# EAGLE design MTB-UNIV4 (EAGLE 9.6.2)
Assembly variants: PFH, SVORK
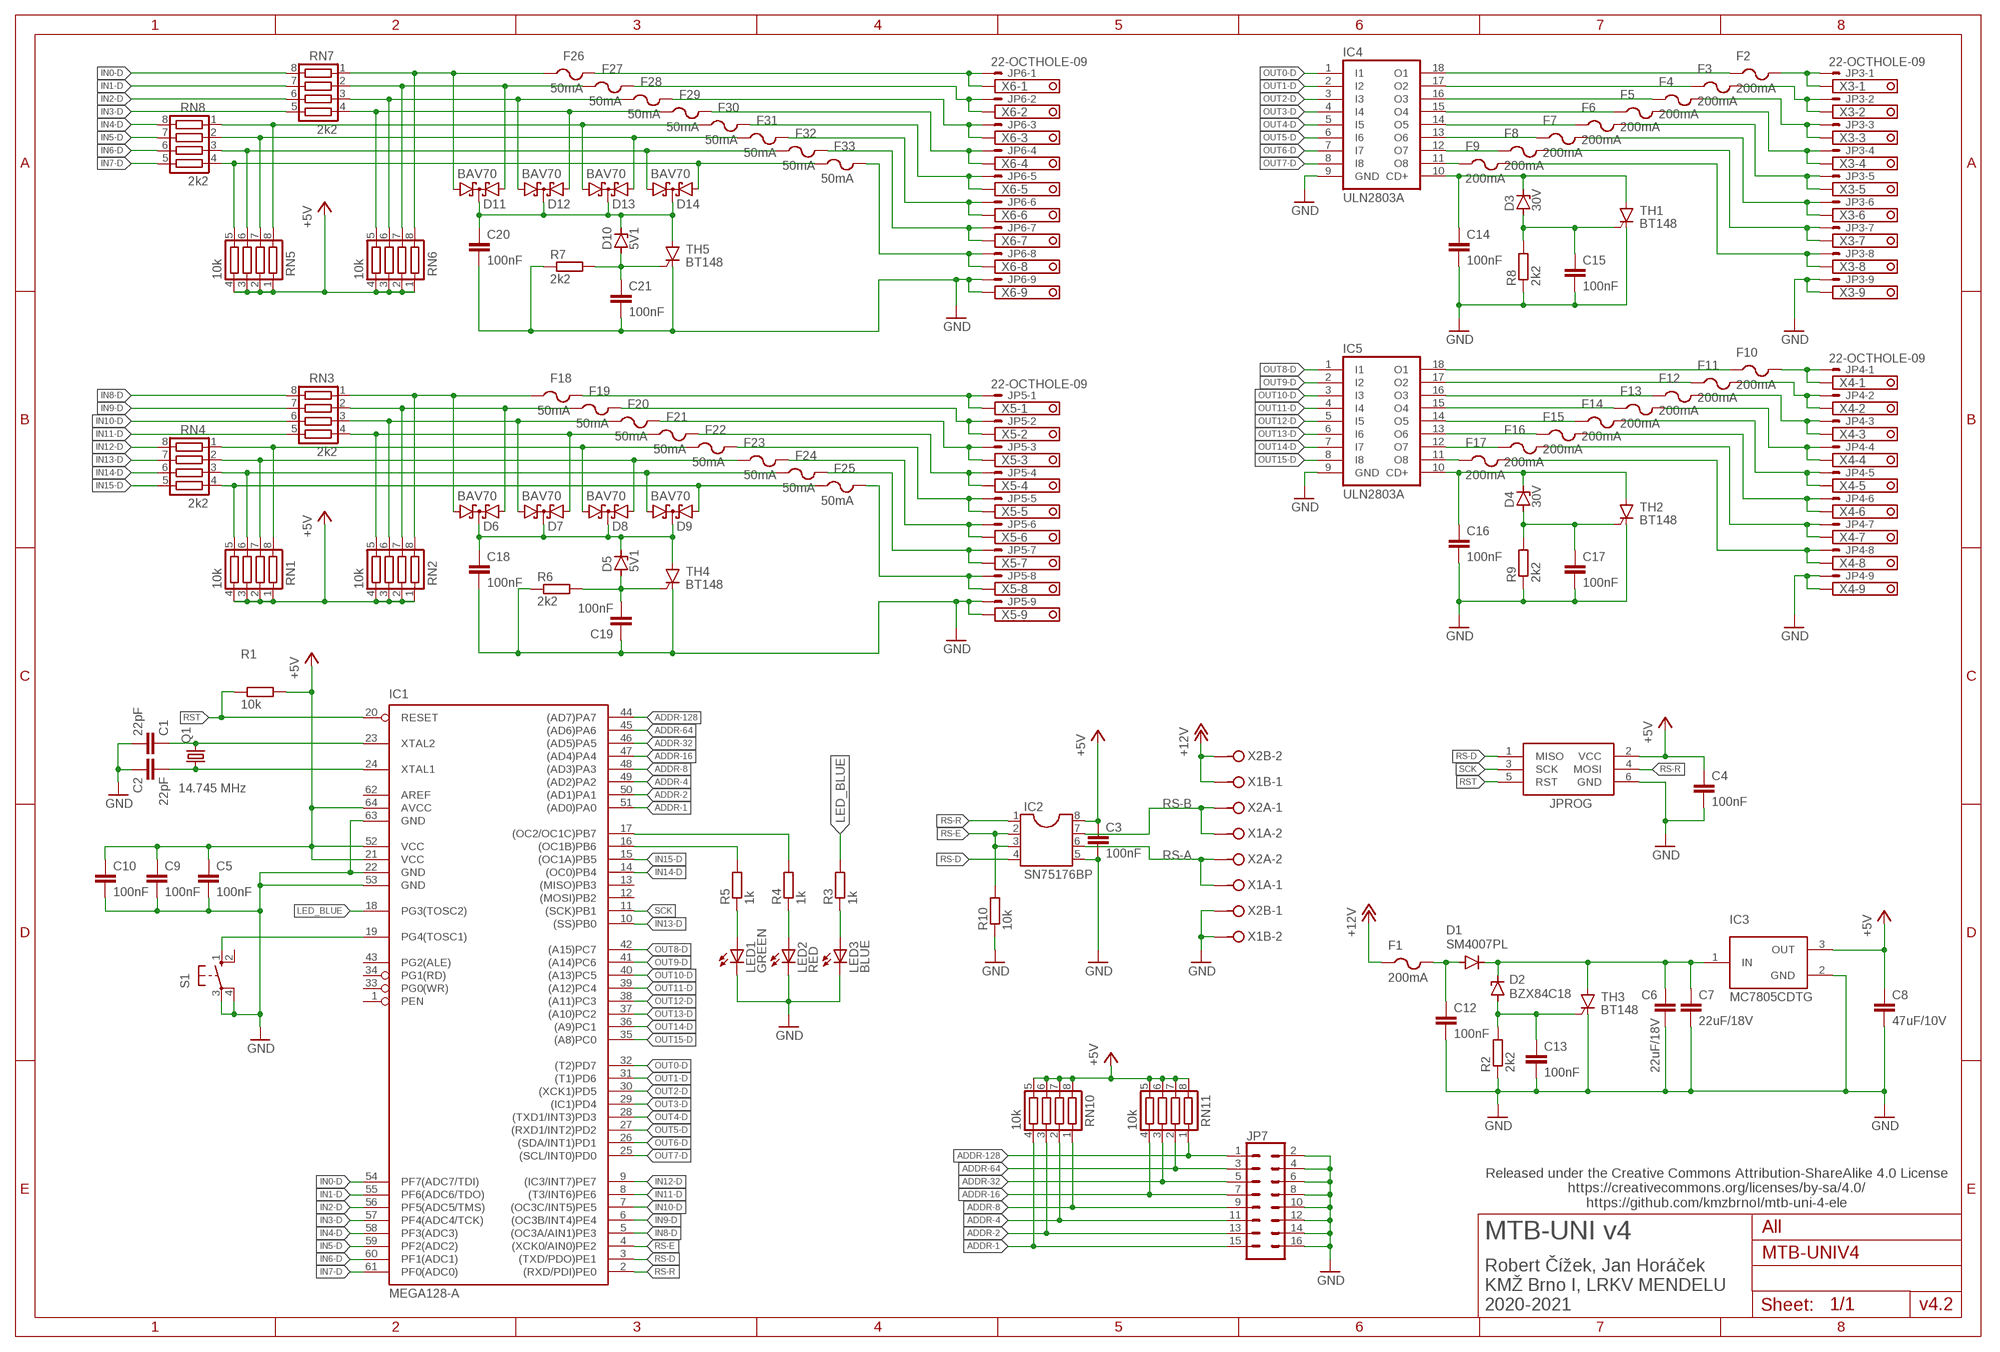
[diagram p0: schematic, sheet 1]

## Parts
C1  22pF  C-EUC0805  [C0805]
C2  22pF  C-EUC0805  [C0805]
C3  100nF  C-EUC0805  [C0805]
C4  100nF  C-EUC0805  [C0805]
C5  100nF  C-EUC0805  [C0805]
C6  22uF/18V  C-EUC0805  [C0805]
C7  22uF/18V  C-EUC1206  [C1206]
C8  47uF/10V  C-EUC1206  [C1206]
C9  100nF  C-EUC0805  [C0805]
C10  100nF  C-EUC0805  [C0805]
C12  100nF  C-EUC0805  [C0805]
C13  100nF  C-EUC0805  [C0805]
C14  100nF  C-EUC0805  [C0805]
C15  100nF  C-EUC0805  [C0805]
C16  100nF  C-EUC0805  [C0805]
C17  100nF  C-EUC0805  [C0805]
C18  100nF  C-EUC0805  [C0805]
C19  100nF  C-EUC0805  [C0805]
C20  100nF  C-EUC0805  [C0805]
C21  100nF  C-EUC0805  [C0805]
D1  SM4007PL  CGRM4007-G  [SOD-123_MINI-SMA]
D2  BZX84C18  ZENER-DIODESOT23  [SOT23]
D3  30V  ZENER-DIODESOT23  [SOT23]
D4  30V  ZENER-DIODESOT23  [SOT23]
D5  5V1  ZENER-DIODESOT23  [SOT23]
D6  BAV70  BAT54C  [SOT23]
D7  BAV70  BAT54C  [SOT23]
D8  BAV70  BAT54C  [SOT23]
D9  BAV70  BAT54C  [SOT23]
D10  5V1  ZENER-DIODESOT23  [SOT23]
D11  BAV70  BAT54C  [SOT23]
D12  BAV70  BAT54C  [SOT23]
D13  BAV70  BAT54C  [SOT23]
D14  BAV70  BAT54C  [SOT23]
F1  200mA  PTCFUSE-1206  [R1206]
F2  200mA  PTCFUSE-1206S  [R1206S]
F3  200mA  PTCFUSE-1206S  [R1206S]
F4  200mA  PTCFUSE-1206S  [R1206S]
F5  200mA  PTCFUSE-1206S  [R1206S]
F6  200mA  PTCFUSE-1206S  [R1206S]
F7  200mA  PTCFUSE-1206S  [R1206S]
F8  200mA  PTCFUSE-1206S  [R1206S]
F9  200mA  PTCFUSE-1206S  [R1206S]
F10  200mA  PTCFUSE-1206S  [R1206S]
F11  200mA  PTCFUSE-1206S  [R1206S]
F12  200mA  PTCFUSE-1206S  [R1206S]
F13  200mA  PTCFUSE-1206S  [R1206S]
F14  200mA  PTCFUSE-1206S  [R1206S]
F15  200mA  PTCFUSE-1206S  [R1206S]
F16  200mA  PTCFUSE-1206S  [R1206S]
F17  200mA  PTCFUSE-1206S  [R1206S]
F18  50mA  PTCFUSE-1206S  [R1206S]
F19  50mA  PTCFUSE-1206S  [R1206S]
F20  50mA  PTCFUSE-1206S  [R1206S]
F21  50mA  PTCFUSE-1206S  [R1206S]
F22  50mA  PTCFUSE-1206S  [R1206S]
F23  50mA  PTCFUSE-1206S  [R1206S]
F24  50mA  PTCFUSE-1206S  [R1206S]
F25  50mA  PTCFUSE-1206S  [R1206S]
F26  50mA  PTCFUSE-1206S  [R1206S]
F27  50mA  PTCFUSE-1206S  [R1206S]
F28  50mA  PTCFUSE-1206S  [R1206S]
F29  50mA  PTCFUSE-1206S  [R1206S]
F30  50mA  PTCFUSE-1206S  [R1206S]
F31  50mA  PTCFUSE-1206S  [R1206S]
F32  50mA  PTCFUSE-1206S  [R1206S]
F33  50mA  PTCFUSE-1206S  [R1206S]
IC1  MEGA128-A  [TQFP64]
IC2  SN75176BP  DIL8  [DIL08]
IC3  MC7805CDTG  MC78M05BDTRKG  [MC78M05BDTRKG]
IC4  ULN2803A  [DIL18]
IC5  ULN2803A  [DIL18]
JP3  22-OCTHOLE-09  [7395-09-OCTHOLE]  (not fitted in variant SVORK)
JP4  22-OCTHOLE-09  [7395-09-OCTHOLE]  (not fitted in variant SVORK)
JP5  22-OCTHOLE-09  [7395-09-OCTHOLE]  (not fitted in variant SVORK)
JP6  22-OCTHOLE-09  [7395-09-OCTHOLE]  (not fitted in variant SVORK)
JP7  CONN_08X2  [2X8]
JPROG  AVRISP-6  [AVRISP]
LED1  GREEN  LEDCHIPLED_0805  [CHIPLED_0805]
LED2  RED  LEDCHIPLED_0805  [CHIPLED_0805]
LED3  BLUE  LEDCHIPLED_0805  [CHIPLED_0805]
Q1  14.745 MHz  CRYSTALHC49UP  [HC49UP]
R1  10k  R-EU_R0805  [R0805]
R2  2k2  R-EU_R0805  [R0805]
R3  1k  R-EU_R0805  [R0805]
R4  1k  R-EU_R0805  [R0805]
R5  1k  R-EU_R0805  [R0805]
R6  2k2  R-EU_R0805  [R0805]
R7  2k2  R-EU_R0805  [R0805]
R8  2k2  R-EU_R0805  [R0805]
R9  2k2  R-EU_R0805  [R0805]
R10  10k  R-EU_R0805  [R0805]
RN1  10k  CTS742C083  [CTS742C083]
RN2  10k  CTS742C083  [CTS742C083]
RN3  2k2  CTS742C083  [CTS742C083]
RN4  2k2  CTS742C083  [CTS742C083]
RN5  10k  CTS742C083  [CTS742C083]
RN6  10k  CTS742C083  [CTS742C083]
RN7  2k2  CTS742C083  [CTS742C083]
RN8  2k2  CTS742C083  [CTS742C083]
RN10  10k  CTS742C083  [CTS742C083]
RN11  10k  CTS742C083  [CTS742C083]
S1  10-XX  [B3F-10XX]
TH1  BT148  [SOT223]
TH2  BT148  [SOT223]
TH3  BT148  [SOT223]
TH4  BT148  [SOT223]
TH5  BT148  [SOT223]
X1A  MVE252-5-V  [MVE252-5-V]
X1B  MVE252-5-V  [MVE252-5-V]
X2A  MVE252-5-V  [MVE252-5-V]
X2B  MVE252-5-V  [MVE252-5-V]
X3  1751316  [1751316]  (not fitted in variant PFH)
X4  1751316  [1751316]  (not fitted in variant PFH)
X5  1751316  [1751316]  (not fitted in variant PFH)
X6  1751316  [1751316]  (not fitted in variant PFH)

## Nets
+5V [power5V]: C3.1 C4.1 C5.1 C8.1 C9.1 C10.1 IC1.21(VCC) IC1.52(VCC) IC1.64(AVCC) IC2.8 IC3.3(OUT) JPROG.2(VCC) R1.2 RN1.1 RN1.2 RN1.3 RN1.4 RN2.1 RN2.2 RN2.3 RN2.4 RN5.1 RN5.2 RN5.3 RN5.4 RN6.1 RN6.2 RN6.3 RN6.4 RN10.5 RN10.6 RN10.7 RN10.8 RN11.5 RN11.6 RN11.7 RN11.8
+12V [power12V]: F1.1 X1B.1 X2B.2
+12V-IN: C6.1 C7.1 D1.C D2.3(C) IC3.1(IN) TH3.2(A)
+12V_MIN: C12.1 D1.A F1.2
ADDR-1: IC1.51((AD0)PA0) JP7.15 RN10.4
ADDR-2: IC1.50((AD1)PA1) JP7.13 RN10.3
ADDR-4: IC1.49((AD2)PA2) JP7.11 RN10.2
ADDR-8: IC1.48((AD3)PA3) JP7.9 RN10.1
ADDR-16: IC1.47((AD4)PA4) JP7.7 RN11.4
ADDR-32: IC1.46((AD5)PA5) JP7.5 RN11.3
ADDR-64: IC1.45((AD6)PA6) JP7.3 RN11.2
ADDR-128: IC1.44((AD7)PA7) JP7.1 RN11.1
BTN: IC1.19(PG4(TOSC1)) S1.1(S)
GND: C1.2 C2.1 C3.2 C4.2 C5.2 C6.2 C7.2 C8.2 C9.2 C10.2 C12.2 C13.2 C14.2 C15.2 C16.2 C17.2 C18.2 C19.1 C20.2 C21.2 IC1.22(GND) IC1.53(GND) IC1.63(GND) IC2.5 IC3.2(GND) IC4.9(GND) IC5.9(GND) JP3.9 JP4.9 JP5.9 JP6.9 JP7.2 JP7.4 JP7.6 JP7.8 JP7.10 JP7.12 JP7.14 JP7.16 JPROG.6(GND) LED1.C LED2.C LED3.C R2.1 R6.1 R7.1 R8.1 R9.1 R10.1 S1.3(P) S1.4(P1) TH1.1(C) TH2.1(C) TH3.1(C) TH4.1(C) TH5.1(C) X1B.2 X2B.1 X3.9 X4.9 X5.9 X6.9
IN0-D: IC1.54(PF7(ADC7/TDI)) RN7.8
IN0-R [io_power]: F26.2 JP6.1 X6.1
IN0-U: D11.1(A1) F26.1 RN6.8 RN7.1
IN1-D: IC1.55(PF6(ADC6/TDO)) RN7.7
IN1-R [io_power]: F27.2 JP6.2 X6.2
IN1-U: D11.2(A2) F27.1 RN6.7 RN7.2
IN2-D: IC1.56(PF5(ADC5/TMS)) RN7.6
IN2-R [io_power]: F28.2 JP6.3 X6.3
IN2-U: D12.1(A1) F28.1 RN6.6 RN7.3
IN3-D: IC1.57(PF4(ADC4/TCK)) RN7.5
IN3-R [io_power]: F29.2 JP6.4 X6.4
IN3-U: D12.2(A2) F29.1 RN6.5 RN7.4
IN4-D: IC1.58(PF3(ADC3)) RN8.8
IN4-R [io_power]: F30.2 JP6.5 X6.5
IN4-U: D13.1(A1) F30.1 RN5.8 RN8.1
IN5-D: IC1.59(PF2(ADC2)) RN8.7
IN5-R [io_power]: F31.2 JP6.6 X6.6
IN5-U: D13.2(A2) F31.1 RN5.7 RN8.2
IN6-D: IC1.60(PF1(ADC1)) RN8.6
IN6-R [io_power]: F32.2 JP6.7 X6.7
IN6-U: D14.1(A1) F32.1 RN5.6 RN8.3
IN7-D: IC1.61(PF0(ADC0)) RN8.5
IN7-R [io_power]: F33.2 JP6.8 X6.8
IN7-U: D14.2(A2) F33.1 RN5.5 RN8.4
IN8-D: IC1.5((OC3A/AIN1)PE3) RN3.8
IN8-R [io_power]: F18.2 JP5.1 X5.1
IN8-U: D6.1(A1) F18.1 RN2.8 RN3.1
IN9-D: IC1.6((OC3B/INT4)PE4) RN3.7
IN9-R [io_power]: F19.2 JP5.2 X5.2
IN9-U: D6.2(A2) F19.1 RN2.7 RN3.2
IN10-D: IC1.7((OC3C/INT5)PE5) RN3.6
IN10-R [io_power]: F20.2 JP5.3 X5.3
IN10-U: D7.1(A1) F20.1 RN2.6 RN3.3
IN11-D: IC1.8((T3/INT6)PE6) RN3.5
IN11-R [io_power]: F21.2 JP5.4 X5.4
IN11-U: D7.2(A2) F21.1 RN2.5 RN3.4
IN12-D: IC1.9((IC3/INT7)PE7) RN4.8
IN12-R [io_power]: F22.2 JP5.5 X5.5
IN12-U: D8.1(A1) F22.1 RN1.8 RN4.1
IN13-D: IC1.10((SS)PB0) RN4.7
IN13-R [io_power]: F23.2 JP5.6 X5.6
IN13-U: D8.2(A2) F23.1 RN1.7 RN4.2
IN14-D: IC1.14((OC0)PB4) RN4.6
IN14-R [io_power]: F24.2 JP5.7 X5.7
IN14-U: D9.1(A1) F24.1 RN1.6 RN4.3
IN15-D: IC1.15((OC1A)PB5) RN4.5
IN15-R [io_power]: F25.2 JP5.8 X5.8
IN15-U: D9.2(A2) F25.1 RN1.5 RN4.4
LED_BLUE: IC1.18(PG3(TOSC2)) R3.2
LED_GREEN: IC1.16((OC1B)PB6) R5.2
LED_RED: IC1.17((OC2/OC1C)PB7) R4.2
N$11: C16.1 D4.3(C) IC5.10(CD+) TH2.2(A)
N$37: C14.1 D3.3(C) IC4.10(CD+) TH1.2(A)
N$46: C15.1 D3.1(A) R8.2 TH1.3(G)
N$56: C17.1 D4.1(A) R9.2 TH2.3(G)
N$57: C13.1 D2.1(A) R2.2 TH3.3(G)
N$60: LED2.A R4.1
N$61: LED1.A R5.1
N$64: LED3.A R3.1
N$70: C18.1 D5.3(C) D6.3(CC) D7.3(CC) D8.3(CC) D9.3(CC) TH4.2(A)
N$71: C19.2 D5.1(A) R6.2 TH4.3(G)
N$80: C20.1 D10.3(C) D11.3(CC) D12.3(CC) D13.3(CC) D14.3(CC) TH5.2(A)
N$81: C21.1 D10.1(A) R7.2 TH5.3(G)
OUT0-D: IC1.32((T2)PD7) IC4.1(I1)
OUT0-R [io_power]: F2.2 JP3.1 X3.1
OUT0-U [io_power]: F2.1 IC4.18(O1)
OUT1-D: IC1.31((T1)PD6) IC4.2(I2)
OUT1-R [io_power]: F3.2 JP3.2 X3.2
OUT2-D: IC1.30((XCK1)PD5) IC4.3(I3)
OUT2-R [io_power]: F4.2 JP3.3 X3.3
OUT2-U [io_power]: F4.1 IC4.16(O3)
OUT3-D: IC1.29((IC1)PD4) IC4.4(I4)
OUT3-R [io_power]: F5.2 JP3.4 X3.4
OUT3-U [io_power]: F5.1 IC4.15(O4)
OUT4-D: IC1.28((TXD1/INT3)PD3) IC4.5(I5)
OUT4-R [io_power]: F6.2 JP3.5 X3.5
OUT4-U [io_power]: F6.1 IC4.14(O5)
OUT5-D: IC1.27((RXD1/INT2)PD2) IC4.6(I6)
OUT5-R [io_power]: F7.2 JP3.6 X3.6
OUT5-U [io_power]: F7.1 IC4.13(O6)
OUT6-D: IC1.26((SDA/INT1)PD1) IC4.7(I7)
OUT6-R [io_power]: F8.2 JP3.7 X3.7
OUT6-U [io_power]: F8.1 IC4.12(O7)
OUT7-D: IC1.25((SCL/INT0)PD0) IC4.8(I8)
OUT7-R [io_power]: F9.2 JP3.8 X3.8
OUT7-U [io_power]: F9.1 IC4.11(O8)
OUT8-D: IC1.42((A15)PC7) IC5.1(I1)
OUT8-R [io_power]: F10.2 JP4.1 X4.1
OUT8-U [io_power]: F10.1 IC5.18(O1)
OUT9-D: IC1.41((A14)PC6) IC5.2(I2)
OUT9-R [io_power]: F11.2 JP4.2 X4.2
OUT9-U [io_power]: F11.1 IC5.17(O2)
OUT10-D: IC1.40((A13)PC5) IC5.3(I3)
OUT10-R [io_power]: F12.2 JP4.3 X4.3
OUT10-U [io_power]: F12.1 IC5.16(O3)
OUT11-D: IC1.39((A12)PC4) IC5.4(I4)
OUT11-R [io_power]: F13.2 JP4.4 X4.4
OUT11-U [io_power]: F13.1 IC5.15(O4)
OUT12-D: IC1.38((A11)PC3) IC5.5(I5)
OUT12-R [io_power]: F14.2 JP4.5 X4.5
OUT12-U [io_power]: F14.1 IC5.14(O5)
OUT13-D: IC1.37((A10)PC2) IC5.6(I6)
OUT13-R [io_power]: F15.2 JP4.6 X4.6
OUT13-U [io_power]: F15.1 IC5.13(O6)
OUT14-D: IC1.36((A9)PC1) IC5.7(I7)
OUT14-R [io_power]: F16.2 JP4.7 X4.7
OUT14-U [io_power]: F16.1 IC5.12(O7)
OUT15-D: IC1.35((A8)PC0) IC5.8(I8)
OUT15-R [io_power]: F17.2 JP4.8 X4.8
OUT15-U [io_power]: F17.1 IC5.11(O8)
OUT-1U [io_power]: F3.1 IC4.17(O2)
RS-A: IC2.6 X1A.1 X2A.2
RS-B: IC2.7 X1A.2 X2A.1
RS-D: IC1.3((TXD/PDO)PE1) IC2.4 JPROG.1(MISO)
RS-E: IC1.4((XCK0/AIN0)PE2) IC2.2 IC2.3 R10.2
RS-R: IC1.2((RXD/PDI)PE0) IC2.1 JPROG.4(MOSI)
RST: IC1.20(RESET) JPROG.5(RST) R1.1
SCK: IC1.11((SCK)PB1) JPROG.3(SCK)
XTAL1: C2.2 IC1.24(XTAL1) Q1.1
XTAL2: C1.1 IC1.23(XTAL2) Q1.2
Unconnected: IC1.1(PEN) IC1.12((MOSI)PB2) IC1.13((MISO)PB3) IC1.33(PG0(WR)) IC1.34(PG1(RD)) IC1.43(PG2(ALE)) IC1.62(AREF) S1.2(S1)

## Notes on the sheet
- Released under the Creative Commons Attribution-ShareAlike 4.0 License
  https://creativecommons.org/licenses/by-sa/4.0/
  https://github.com/kmzbrnoI/mtb-uni-4-ele
- All
- MTB-UNI v4
- Robert Čížek, Jan Horáček
  KMŽ Brno I, LRKV MENDELU
  2020-2021
- v4.2

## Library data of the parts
C1 C2 = rcl:C-EU: CAPACITOR, European symbol; LCSC_PART: C1804
C3 C4 C12 C15-C19 C21 = rcl:C-EU: CAPACITOR, European symbol; LCSC_PART: C49678
C5 C7 C10 = rcl:C-EU: CAPACITOR, European symbol
C6 = rcl:C-EU: CAPACITOR, European symbol; LCSC_PART: C45783
C8 = rcl:C-EU: CAPACITOR, European symbol; LCSC_PART: C96123
C9 C13 C14 = rcl:C-EU: CAPACITOR, European symbol; LCSC_PART: C68978
C20 = rcl:C-EU: CAPACITOR, European symbol; LCSC_PART: C24497
D1 = diode:CGRM400*-G: Molded plasitc,JEDEC SOD-123/Mini SMA; LCSC_PART: C64898
D2 = diode:ZENER-DIODE: Z-Diode
D3 D4 = diode:ZENER-DIODE: Z-Diode; LCSC_PART: C353849
D5 D10 = diode:ZENER-DIODE: Z-Diode; LCSC_PART: C294621
D6-D9 D11-D14 = diode:BAT54C: Schottky Diodes Source: Fairchild .. BAT54.pdf; LCSC_PART: C68978
F1-F17 = adafruit_edited:PTCFUSE: PTC fuses, resettable thermistors; LCSC_PART: C70067
F18-F25 F27-F33 = adafruit_edited:PTCFUSE: PTC fuses, resettable thermistors; LCSC_PART: C261946
F26 = adafruit_edited:PTCFUSE: PTC fuses, resettable thermistors; LSCS_PART: C261946
IC1 = atmel:MEGA128: MICROCONTROLLER 128 Kbytes FLASH 4 Kbytes SRAM 4 Kbytes EEPROM DUAL USART 8-channel 10 bit ADC Source: avr.lbr; LCSC_PART: C6510; MPN: ATMEGA128-16AU; OC_FARNELL: 9171118; OC_NEWARK: 95K7364
IC2 = ic-package:DIL8: Dual In Line / Socket
IC3 = LDO:MC78M05BDTRKG: IC REG LINEAR 5V 500MA DPAK Manufacturer's datasheet; CREATED_BY: PCBLayout.com; DIGIKEY_PN: MC78M05BDTRKGOSCT-ND; LCSC_PART: C58069; MANUFACTURER: ON Semiconductor; MPN: IC REG LINEAR 5V 500MA DPAK; PACKAGE: DPak
IC4 IC5 = uln-udn:ULN2803A: DRIVER ARRAY
JP3-JP6 = con-molex:22-?-09: CONNECTOR wire to board 2.54 mm (.1 inch) pitch header
JP7 = SparkFun-Connectors:CONN_08X2: Multi connection point. Often used as Generic Header-pin footprint for 0.1 inch spaced/style header connections You can populate with any combo of single row headers, but if you'd like an exact match, check this: Header - 2x8 (Male, 0.1") (PRT-13156) On any of the 0.1 inch spaced packages, you can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
JPROG = adafruit:AVRISP: AVR ISP HEADER Standard 6 pin header for AVR programming
LED1-LED3 = adafruit:LED: LED
Q1 = crystal:CRYSTAL: CRYSTAL; OC_FARNELL: unknown; OC_NEWARK: unknown
R1 R10 = rcl:R-EU_: RESISTOR, European symbol; LCSC_PART: C17513
R2 R6-R9 = rcl:R-EU_: RESISTOR, European symbol; LCSC_PART: C17520
R3-R5 = rcl:R-EU_: RESISTOR, European symbol
RN1 RN5 RN6 RN10 RN11 = resistor-net:CTS742C083: Chip Resistor Array 4 Single Resistor Source: http://www.ctscorp.com/components/Datasheets/CTSChipArrayDs.pdf; LCSC_PART: C29718; OC_FARNELL: unknown; OC_NEWARK: unknown
RN2 = resistor-net:CTS742C083: Chip Resistor Array 4 Single Resistor Source: http://www.ctscorp.com/components/Datasheets/CTSChipArrayDs.pdf; LCSC_PART: C29718; OC_FARNELL: unknown; OC_NEWARK: unknown; SPICEPREFIX: X
RN3 RN4 RN7 RN8 = resistor-net:CTS742C083: Chip Resistor Array 4 Single Resistor Source: http://www.ctscorp.com/components/Datasheets/CTSChipArrayDs.pdf; LCSC_PART: C12001; OC_FARNELL: unknown; OC_NEWARK: unknown
S1 = switch-omron:10-XX: OMRON SWITCH; MPN: B3F-1000; OC_FARNELL: 176432; OC_NEWARK: 36M3542
TH1-TH5 = ElectroKrt:BT148
X1A X1B X2A X2B = con-malina:MVE252-5-V
X3-X6 = con-phoenix-350:1751316: MKDS 1/ 9-3,5 Printklemme Nennstrom: 10 A Bemessungsspannung: 160 V Raster: 3,5 mm Polzahl: 9 Montageart: Löten Anschlussart: Schraubanschluss Anschlussrichtung vom Leiter zur Platine: 0° Source: http://eshop.phoenixcontact.com .. 1751316.pdf; OC_FARNELL: unknown; OC_NEWARK: unknown

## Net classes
0 default: width 0.305 mm
1 mountpad: clearance 1 mm to class 0, clearance 1 mm
2 io_power: width 0.813 mm
3 power5V: width 0.406 mm
4 power12V: width 0.406 mm, clearance 1 mm to class 0, clearance 1 mm to class 1, clearance 1 mm to class 2, clearance 1 mm to class 3

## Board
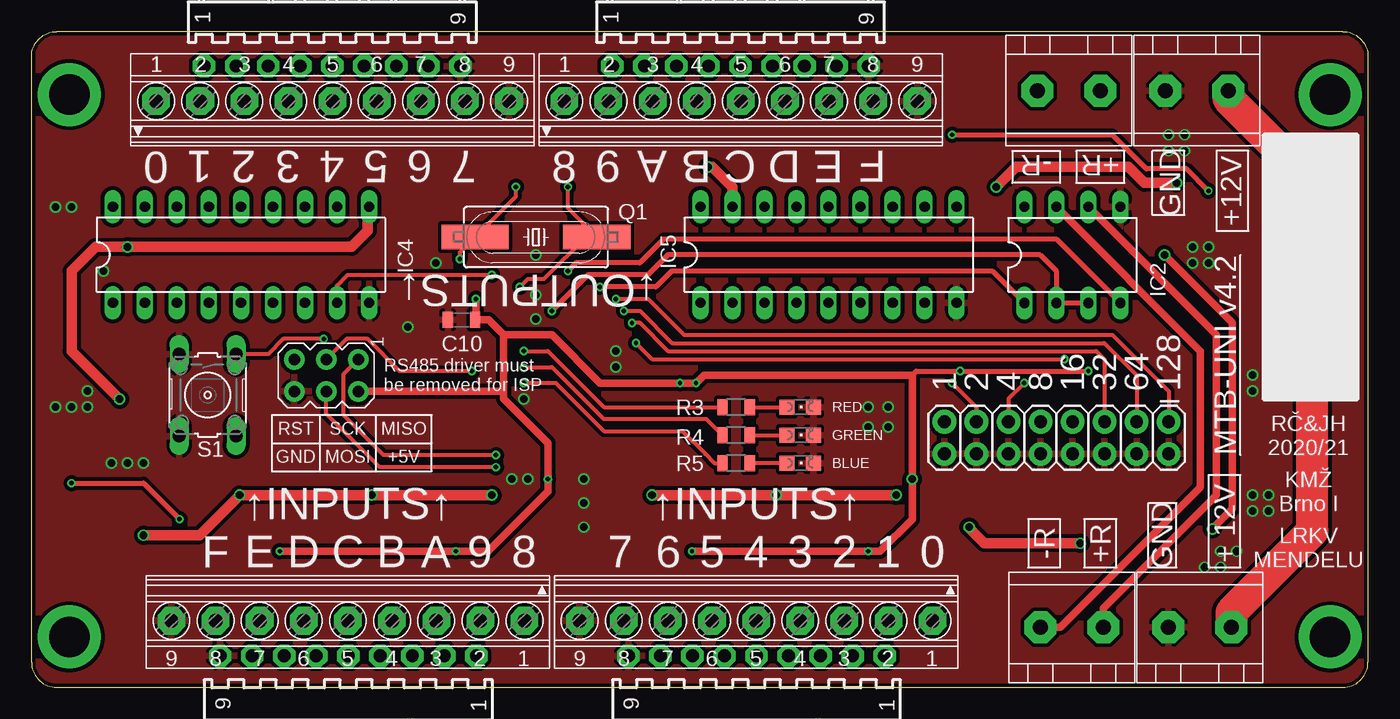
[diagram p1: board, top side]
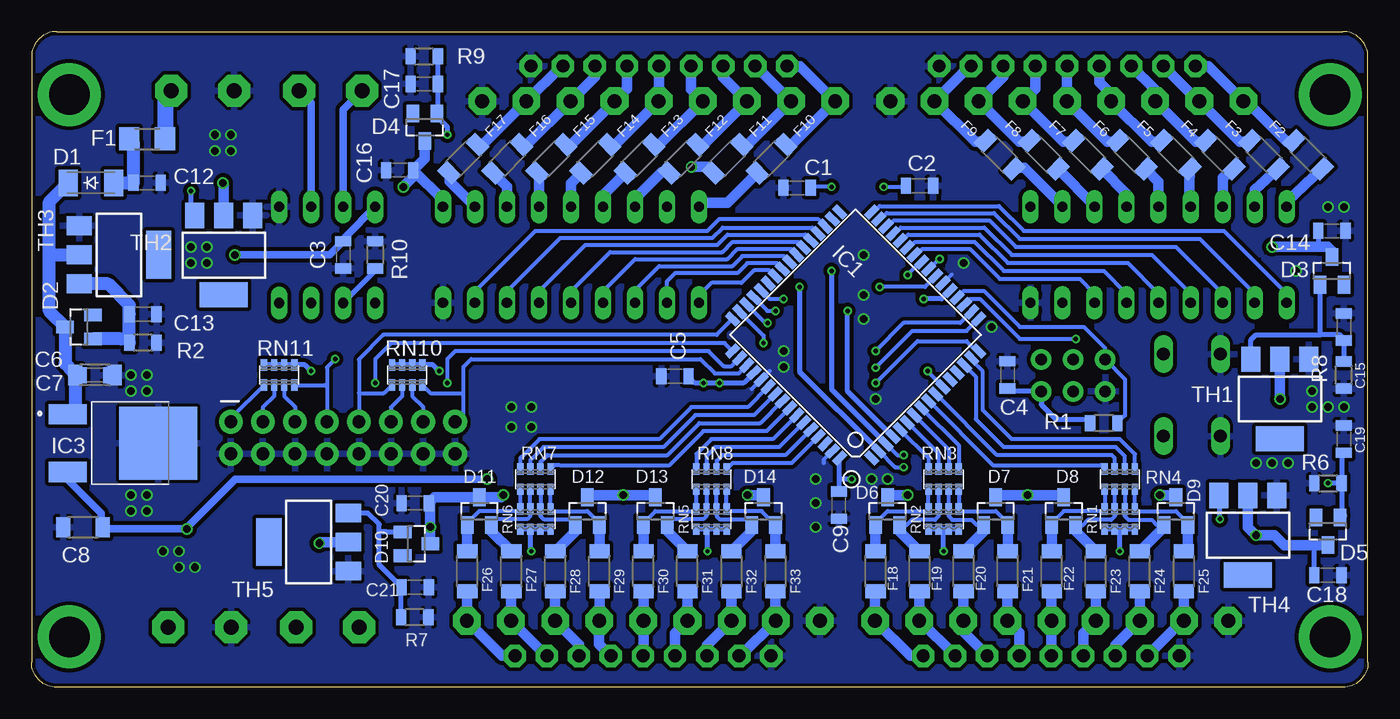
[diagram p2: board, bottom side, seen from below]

Size 106 x 52 mm. Coordinates in mm from the lower left corner, seen from the top.
Outline: 2,0 104,0 arc90 106,2 106,50 arc90 104,52 2,52 arc90 0,50 0,2 arc90 2,0
Copper layers (1*16): Top 0.035mm / dielectric 1.5mm / Bottom 0.035mm
Design rules "SeeedStudio_2layer_DRU_no_angle_20140221": minimum track width 6mil, minimum drill 12mil, track to track 6mil, track to pad 6mil, pad to pad 6mil, via to via 6mil, smd to smd 0mil, copper to edge 10mil, drill to drill 10mil, minimum pad ring 10mil, minimum via ring 6mil, stop-mask expansion 2mil, vias tented up to drill 100mil, thermal gap 10mil

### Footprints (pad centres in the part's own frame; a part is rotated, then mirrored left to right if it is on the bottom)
C0805 = smd 0.813 x 1.27: 1 -1.077,0; 2 1.077,0
C1206 = smd 1.1 x 1.6: 1 -1.577,0; 2 1.577,0
SOD-123_MINI-SMA = smd 1.5 x 2.1: A 1.8,0; C -1.8,0
SOT23 = smd 1 x 1.4: 1 -0.95,-1.1; 2 0.95,-1.1; 3 0,1.1
R1206 = smd 1.6 x 1.803: 1 -1.422,0; 2 1.422,0
R1206S = smd 1.1 x 1.6: 1 -1.577,0; 2 1.577,0
TQFP64 = smd 1.194 x 0.559: 1 -7.8,6; 2 -7.8,5.2; 3 -7.8,4.4; 4 -7.8,3.6; 5 -7.8,2.8; 6 -7.8,2; 7 -7.8,1.2; 8 -7.8,0.4; 9 -7.8,-0.4; 10 -7.8,-1.2; 11 -7.8,-2; 12 -7.8,-2.8; 13 -7.8,-3.6; 14 -7.8,-4.4; 15 -7.8,-5.2; 16 -7.8,-6; 33 7.8,-6; 34 7.8,-5.2; 35 7.8,-4.4; 36 7.8,-3.6; 37 7.8,-2.8; 38 7.8,-2; 39 7.8,-1.2; 40 7.8,-0.4; 41 7.8,0.4; 42 7.8,1.2; 43 7.8,2; 44 7.8,2.8; 45 7.8,3.6; 46 7.8,4.4; 47 7.8,5.2; 48 7.8,6 | smd 0.559 x 1.194: 17 -6,-7.8; 18 -5.2,-7.8; 19 -4.4,-7.8; 20 -3.6,-7.8; 21 -2.8,-7.8; 22 -2,-7.8; 23 -1.2,-7.8; 24 -0.4,-7.8; 25 0.4,-7.8; 26 1.2,-7.8; 27 2,-7.8; 28 2.8,-7.8; 29 3.6,-7.8; 30 4.4,-7.8; 31 5.2,-7.8; 32 6,-7.8; 49 6,7.8; 50 5.2,7.8; 51 4.4,7.8; 52 3.6,7.8; 53 2.8,7.8; 54 2,7.8; 55 1.2,7.8; 56 0.4,7.8; 57 -0.4,7.8; 58 -1.2,7.8; 59 -2,7.8; 60 -2.8,7.8; 61 -3.6,7.8; 62 -4.4,7.8; 63 -5.2,7.8; 64 -6,7.8
DIL08 = drill 0.813 long: 1 -3.81,-3.81; 2 -1.27,-3.81; 3 1.27,-3.81; 4 3.81,-3.81; 5 3.81,3.81; 6 1.27,3.81; 7 -1.27,3.81; 8 -3.81,3.81
MC78M05BDTRKG = smd 1.6 x 3: 1 -2.285,-4.08; 3 2.285,-4.08 | smd 5.8 x 6.2: 2 0,3.1
DIL18 = drill 0.813 long: 1 -10.16,-3.81; 2 -7.62,-3.81; 3 -5.08,-3.81; 4 -2.54,-3.81; 5 0,-3.81; 6 2.54,-3.81; 7 5.08,-3.81; 8 7.62,-3.81; 9 10.16,-3.81; 10 10.16,3.81; 11 7.62,3.81; 12 5.08,3.81; 13 2.54,3.81; 14 0,3.81; 15 -2.54,3.81; 16 -5.08,3.81; 17 -7.62,3.81; 18 -10.16,3.81
7395-09-OCTHOLE = drill 1.016 pad 1.778 octagon: 1 10.16,0; 2 7.62,0; 3 5.08,0; 4 2.54,0; 5 0,0; 6 -2.54,0; 7 -5.08,0; 8 -7.62,0; 9 -10.16,0
2X8 = drill 1.016 pad 1.88: 1 0,0; 2 0,2.54; 3 2.54,0; 4 2.54,2.54; 5 5.08,0; 6 5.08,2.54; 7 7.62,0; 8 7.62,2.54; 9 10.16,0; 10 10.16,2.54; 11 12.7,0; 12 12.7,2.54; 13 15.24,0; 14 15.24,2.54; 15 17.78,0; 16 17.78,2.54
AVRISP = drill 0.9 pad 1.626: 1 -1.27,2.54; 2 1.27,2.54; 3 -1.27,0; 4 1.27,0; 5 -1.27,-2.54; 6 1.27,-2.54
CHIPLED_0805 = smd 1.2 x 1.2: A 0,-1.05; C 0,1.05
HC49UP = smd 5.334 x 1.93: 1 -4.826,0; 2 4.826,0
R0805 = smd 0.813 x 1.27: 1 -1.077,0; 2 1.077,0
CTS742C083 = smd 0.5 x 0.9: 1 -1.2,-0.8; 2 -0.4,-0.8; 3 0.4,-0.8; 4 1.2,-0.8; 5 1.2,0.8; 6 0.4,0.8; 7 -0.4,0.8; 8 -1.2,0.8
B3F-10XX = drill 1.016 long: 1 -3.251,2.261; 2 3.251,2.261; 3 -3.251,-2.261; 4 3.251,-2.261
SOT223 = smd 1.5 x 2: 1 -2.3,-3.15; 2 0,-3.15; 3 2.3,-3.15 | smd 3.8 x 2: 4 0,3.15
MVE252-5-V = drill 1.2 pad 2.54 octagon: 1 0,0; 2 5,0
1751316 = drill 1.1 pad 2.184 octagon: 1 -13.973,-0.1; 2 -10.473,-0.1; 3 -6.973,-0.1; 4 -3.473,-0.1; 5 0.028,-0.1; 6 3.527,-0.1; 7 7.027,-0.1; 8 10.527,-0.1; 9 14.027,-0.1

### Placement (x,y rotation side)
C1  45.28,39.6 180 bottom
C2  35.56,39.77 180 bottom
C3  81.28,34.29 270 bottom
C4  28.59,24.77 90 bottom
C5  54.97,24.66 180 bottom
C6  100.97,24.77 0 bottom
C7  100.97,24.77 0 bottom
C8  101.92,12.7 180 bottom
C9  41.97,14.45 270 bottom
C10  34.1,29.14 180 top
C12  96.84,40.01 0 bottom
C13  97.16,29.59 0 bottom
C14  2.86,36.2 0 bottom
C15  1.91,28.57 90 bottom
C16  76.8,41.01 180 bottom
C17  74.86,47.84 180 bottom
C18  3.17,8.89 0 bottom
C19  1.91,19.68 270 bottom
C20  75.56,14.61 180 bottom
C21  75.56,7.94 0 bottom
D1  101.28,40.01 0 bottom
D2  102.23,28.57 90 bottom
D3  2.86,33.02 0 bottom
D4  74.81,44.41 180 bottom
D5  3.17,12.38 180 bottom
D6  38.1,13.97 0 bottom
D7  29.53,13.97 0 bottom
D8  24.13,13.97 0 bottom
D9  15.24,13.97 0 bottom
D10  75.47,11.38 270 bottom
D11  70.48,13.97 0 bottom
D12  61.91,13.97 0 bottom
D13  56.52,13.97 0 bottom
D14  47.94,13.97 0 bottom
F1  96.84,43.5 180 bottom
F2  4.76,42.23 135 bottom
F3  8.26,42.23 135 bottom
F4  11.75,42.23 135 bottom
F5  15.24,42.23 135 bottom
F6  18.73,42.23 135 bottom
F7  22.23,42.23 135 bottom
F8  25.72,42.23 135 bottom
F9  29.21,42.23 135 bottom
F10  47.31,41.91 45 bottom
F11  50.8,41.91 45 bottom
F12  54.29,41.91 45 bottom
F13  57.78,41.91 45 bottom
F14  61.28,41.91 45 bottom
F15  64.77,41.91 45 bottom
F16  68.26,41.91 45 bottom
F17  71.75,41.91 45 bottom
F18  39.05,9.21 270 bottom
F19  35.56,9.21 270 bottom
F20  32.07,9.21 270 bottom
F21  28.57,9.21 270 bottom
F22  25.08,9.21 270 bottom
F23  21.59,9.21 270 bottom
F24  18.1,9.21 270 bottom
F25  14.61,9.21 270 bottom
F26  71.44,9.21 270 bottom
F27  67.94,9.21 270 bottom
F28  64.45,9.21 270 bottom
F29  60.96,9.21 270 bottom
F30  57.47,9.21 270 bottom
F31  53.98,9.21 270 bottom
F32  50.48,9.21 270 bottom
F33  46.99,9.21 270 bottom
IC1  40.64,27.94 135 bottom
IC2  82.55,34.29 0 top
IC3  99.06,19.37 270 bottom
IC4  16.61,34.3 0 top
IC5  63.22,34.3 0 top
JP3  23.85,49.26 180 top
JP4  56.23,49.26 180 top
JP5  25.12,2.5 0 top
JP6  57.5,2.5 0 top
JP7  90.19,21.05 180 top
JPROG  23.38,24.73 270 top
LED1  60.96,17.78 270 top
LED2  60.96,20 270 top
LED3  60.96,22.23 270 top
Q1  40.01,35.7 0 top
R1  20.95,20.95 180 bottom
R2  97.16,27.32 180 bottom
R3  55.88,22.23 180 top
R4  55.88,20 180 top
R5  55.88,17.78 180 top
R6  3.17,16.19 0 bottom
R7  75.61,5.55 180 bottom
R8  1.91,24.77 90 bottom
R9  74.86,50.02 0 bottom
R10  78.74,34.29 270 bottom
RN1  19.68,13.34 0 bottom
RN2  33.66,13.34 0 bottom
RN3  33.66,16.51 0 bottom
RN4  19.68,16.51 0 bottom
RN5  52.07,13.34 0 bottom
RN6  66.04,13.34 0 bottom
RN7  66.04,16.51 0 bottom
RN8  52.07,16.51 0 bottom
RN10  76.2,24.77 0 bottom
RN11  86.36,24.77 0 bottom
S1  13.97,23.18 270 top
TH1  6.99,22.86 180 bottom
TH2  90.75,34.27 180 bottom
TH3  99.06,34.29 270 bottom
TH4  9.53,12.06 180 bottom
TH5  84.03,11.53 90 bottom
X1A  84.77,47.31 180 top
X1B  94.93,47.31 180 top
X2A  80.01,4.76 0 top
X2B  90.17,4.76 0 top
X3  23.85,46.58 0 top
X4  56.23,46.58 0 top
X5  25.12,5.18 180 top
X6  57.5,5.18 180 top

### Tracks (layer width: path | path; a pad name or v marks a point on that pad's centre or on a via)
+5V  (via drill 0.35, 0.6)
  Top 0.406: JPROG.2 25.95,23.5 | 69.85,24.77 70.17,25.08 v73.66,25.08 v83.82,25.08 | v51.44,24.13 v52.7,24.13
  Top 0.61: v35.24,30.8 35.24,29.17 C10.1 36.25,29.14 37.45,27.94 | 25.95,23.5 37.45,23.5 | v89.85,34.29 95.25,28.89 95.25,14.15 v93.66,12.56 | v19.68,10.79 v33.66,10.79 36.2,10.79 40.96,15.56 v40.96,16.51 40.96,19.37 37.45,22.88 37.45,23.5 | v52.39,10.79 v66.36,10.79 67.31,10.79 69.85,13.34 v69.85,16.51 69.85,24.77 53.34,24.77 v52.7,24.13 45.09,24.13 41.27,27.94 37.45,27.94 | 37.45,23.5 37.45,27.94
  Bottom 0.406: IC1.21 33.82,30.8 v35.24,30.8 | C4.1 28.45,23.46 JPROG.2 25.92,22.43 24.77,21.27 22.41,21.27 22.3,21.23 R1.2 | RN11.8 RN11.7 RN11.6 RN11.5 84.3,25.57 v83.82,25.08 | RN10.8 RN10.7 RN10.6 RN10.5 74.14,25.57 v73.66,25.08 | RN1.4 RN1.3 19.68,12.54 | 19.68,12.54 RN1.2 RN1.1 | RN2.4 RN2.3 33.66,12.54 | 33.66,12.54 RN2.2 RN2.1 | v33.66,10.79 33.66,12.54 | v19.68,10.79 19.68,12.54 | RN6.4 RN6.3 RN6.2 | RN6.2 RN6.1 | RN5.4 RN5.3 RN5.2 | RN5.2 RN5.1 | v52.39,10.79 52.39,12.45 RN5.2 | RN6.2 66.44,10.88 v66.36,10.79 | C9.1 41.91,15.58 41.91,16.51 | 41.91,16.51 IC1.64 | IC1.52 49.54,24.13 v52.7,24.13 53.36,24.13 C5.1 | v40.96,16.51 41.91,16.51
  Bottom 0.61: IC2.8 81.1,35.74 C3.1 82.36,34.29 v89.85,34.29 | IC3.3 103.14,16.45 100.48,13.79 100.56,12.79 100.43,12.79 C8.1 100.34,12.57 100.33,12.56 v93.66,12.56 93.66,12.7 89.85,16.51 v69.85,16.51
+12V
  Top 2.54: X2B.2 95.17,5.95 101.6,12.38 101.6,40.01 94.93,46.67 X1B.1
  Bottom 1.27: X1B.1 95.42,46.83 F1.1
+12V-IN
  Bottom 0.61: C6.1 C7.1
  Bottom 1.016: 104.59,34.29 TH3.2 | 104.59,34.29 104.59,29.84 D2.3 103.33,25.68 C7.1 102.54,21.9 102.23,21.59 103.08,21.59 IC3.1 | D1.C 104.59,38.49 104.59,34.29
+12V_MIN
  Bottom 1.016: D1.A C12.1 97.92,43.15 F1.2
ADDR-1
  Bottom 0.305: JP7.15 71.75,21.71 71.75,23.33 | IC1.51 49.9,24.9 51.81,24.9 52.94,26.04 71.12,26.04 71.75,25.4 71.75,23.33 | RN10.4 74.36,23.33 71.75,23.33
ADDR-2  (via drill 0.35)
  Top 0.305: v73.03,24.13 74.95,22.2 JP7.13
  Bottom 0.305: IC1.50 50.47,25.47 51.1,25.47 52.31,26.67 72.39,26.67 73.03,26.04 v73.03,24.13 | RN10.3 75.8,23.09 74.95,22.25 JP7.13
ADDR-4  (via drill 0.35)
  Top 0.305: v78.74,24.13 77.49,22.88 JP7.11
  Bottom 0.305: IC1.49 51.04,27.3 77.47,27.3 78.74,26.04 v78.74,24.13 | RN10.2 76.6,23.09 77.49,22.2 JP7.11
ADDR-8
  Bottom 0.305: IC1.48 51.67,27.94 78.11,27.94 80.03,26.02 80.03,23.33 | 80.03,23.33 JP7.9 | RN10.1 78.03,23.33 80.03,23.33
ADDR-16  (via drill 0.35)
  Top 0.305: v47.94,27.3 49.21,26.04 v81.92,26.04
  Bottom 0.305: IC1.47 47.94,27.89 v47.94,27.3 | 82.57,23.81 82.57,25.38 v81.92,26.04 | 82.57,23.81 JP7.7 | RN11.4 82.72,23.96 82.57,23.81
ADDR-32  (via drill 0.35)
  Top 0.305: v47.62,28.89 48.26,28.89 50.48,26.67 84.45,26.67 85.11,26.02 JP7.5
  Bottom 0.305: IC1.46 47.81,28.89 v47.62,28.89 | RN11.3 85.96,23.09 85.11,22.25 JP7.5
ADDR-64  (via drill 0.35)
  Top 0.305: v46.99,29.84 48.26,29.84 50.8,27.3 85.09,27.3 87.65,24.75 JP7.3
  Bottom 0.305: IC1.45 47.64,29.84 v46.99,29.84 | RN11.2 86.76,23.09 87.65,22.2 JP7.3
ADDR-128  (via drill 0.35)
  Top 0.305: v46.35,30.8 48.9,30.8 51.75,27.94 85.72,27.94 90.19,23.48 JP7.1
  Bottom 0.305: IC1.44 47.46,30.8 v46.35,30.8 | RN11.1 90.19,21.34 JP7.1
BTN  (via drill 0.35)
  Top 0.305: v23.18,27.62 19.96,27.62 18.77,26.43 S1.1
  Bottom 0.305: IC1.19 31.56,30.8 30.8,30.8 27.62,27.62 v23.18,27.62
GND  (via drill 0.6)
  Bottom 0.305: IC1.22 33.02,32.73 | 48.9,23.64 IC1.53 47.46,25.08 | IC1.63 43.18,18.05 43.18,17.78
  other vias: 29.84,28.57 67.94,20.64 67.94,22.23 66.36,20.64 66.36,22.23 96.84,15.24 98.11,15.24 43.81,16.51 43.81,14.61 43.81,12.7 40.01,31.11 40.01,34.29 40.01,29.21 93.34,34.92 92.08,33.66 92.08,34.92 93.34,33.66 32.07,33.66 98.11,13.97 96.84,13.97 96.84,23.5 96.84,24.77 98.11,23.5 98.11,24.77 4.45,22.23 4.45,23.5 3.17,22.23 5.71,33.02 3.17,38.1 1.91,38.1 1.91,22.23 8.89,17.78 7.62,17.78 6.35,17.78 91.44,42.55 90.17,42.55 90.17,43.81 91.44,43.81 95.57,10.79 94.3,10.79 94.3,9.53 93.03,9.53 39.37,16.51 38.1,16.51 46.35,25.4 46.35,26.67 39.05,22.86
  pour Top (isolate 0.305): -0.33,-0.06 106.19,-0.06 106.19,51.9 -0.33,51.9
  pour Bottom (isolate 0.305): -0.42,-0.28 106.28,-0.28 106.28,51.81 -0.42,51.81
IN0-D
  Bottom 0.305: IC1.54 49.18,22.23 53.66,22.23 56.2,19.68 65.72,19.68 67.15,18.26 67.24,18.17 RN7.8
IN0-R
  Bottom 0.813: JP6.1 68.69,2.5 X6.1 71.47,7.19 F26.2
IN0-U
  Bottom 0.305: RN7.1 RN6.8 67.41,13.97 70.48,13.97 71.44,13.02 D11.1
  Bottom 0.813: D11.1 F26.1
IN1-D
  Bottom 0.305: IC1.55 48.69,21.59 53.34,21.59 55.88,19.05 65.41,19.05 66.36,18.1 66.44,18.02 RN7.7
IN1-R
  Bottom 0.813: JP6.2 65.19,2.5 X6.2 67.97,7.62 F27.2
IN1-U
  Bottom 0.305: RN7.2 RN6.7 66.44,13.57 66.67,13.34 69.85,13.34 69.85,12.69 69.53,12.37
  Bottom 0.813: F27.1 69.53,12.37 D11.2
IN2-D
  Bottom 0.305: IC1.56 48.19,20.95 53.02,20.95 55.56,18.41 65.09,18.41 65.56,17.94 65.64,17.86 RN7.6
IN2-R
  Bottom 0.813: JP6.3 62.58,3.39 X6.3 64.47,7.61 F28.2
IN2-U
  Bottom 0.305: RN7.3 RN6.6 65.64,13.57 65.41,13.34 63.33,13.34 D12.1
  Bottom 0.813: F28.1 62.86,12.37 D12.1
IN3-D
  Bottom 0.305: IC1.57 47.69,20.32 52.7,20.32 55.4,17.63 64.14,17.63 64.52,17.63 RN7.5
IN3-R
  Bottom 0.813: JP6.4 60.97,3.43 X6.4 60.96,5.29 F29.2
IN3-U
  Bottom 0.305: RN7.4 RN6.5 64.67,13.97 61.91,13.97 60.96,13.02 D12.2
  Bottom 0.813: F29.1 D12.2
IN4-D
  Bottom 0.305: IC1.58 47.2,19.68 52.07,19.68 53.27,18.48 RN8.8
IN4-R
  Bottom 0.813: JP6.5 57.47,2.53 X6.5 F30.2
IN4-U
  Bottom 0.305: RN8.1 RN5.8 53.44,13.97 56.52,13.97 57.47,13.02 D13.1
  Bottom 0.813: F30.1 D13.1
IN5-D
  Bottom 0.305: IC1.59 46.7,19.05 51.75,19.05 52.47,18.33 RN8.7
IN5-R
  Bottom 0.813: JP6.6 54.96,4.29 X6.6 53.97,5.71 53.98,5.71 F31.2
IN5-U
  Bottom 0.305: RN8.2 RN5.7 52.47,13.57 52.7,13.34 55.88,13.34 55.88,12.69 55.56,12.37
  Bottom 0.813: F31.1 55.56,12.37 D13.2
IN6-D
  Bottom 0.305: IC1.60 46.2,18.41 51.21,18.41 51.64,17.99 51.67,17.96 RN8.6
IN6-R
  Bottom 0.813: JP6.7 52.42,3.33 X6.7 F32.2
IN6-U
  Bottom 0.305: RN8.3 RN5.6 51.67,13.57 51.44,13.34 48.9,13.34 48.89,13.33 48.89,12.37
  Bottom 0.813: F32.1 48.89,12.37 D14.1
IN7-D
  Bottom 0.305: IC1.61 45.71,17.78 50.16,17.78 50.4,17.78 RN8.5
IN7-R
  Bottom 0.813: JP6.8 49.76,2.5 X6.8 46.99,5.3 46.99,5.71 F33.2
IN7-U
  Bottom 0.305: RN8.4 RN5.5 50.7,13.97 48.09,13.97 D14.2
  Bottom 0.813: F33.1 D14.2
IN8-D
  Bottom 0.305: RN3.8 34.85,18.2 IC1.5
IN8-R
  Bottom 0.813: JP5.1 36.31,2.5 X5.1 39.09,7.56 F18.2
IN8-U
  Bottom 0.305: RN3.1 RN2.8 35.02,13.97 38.1,13.97 39.05,13.02 D6.1
  Bottom 0.813: D6.1 F18.1
IN9-D
  Bottom 0.305: RN3.7 34.05,18.53 34.12,18.59 IC1.6
IN9-R
  Bottom 0.813: JP5.2 35.52,5.28 X5.2 35.59,7.54 F19.2
IN9-U
  Bottom 0.305: RN3.2 RN2.7 34.05,13.57 34.34,13.29 36.18,13.29 36.6,12.87 D6.2
  Bottom 0.813: D6.2 37.15,12.37 F19.1
IN10-D
  Bottom 0.305: RN3.6 33.26,18.86 IC1.7
IN10-R
  Bottom 0.813: JP5.3 32.09,4.39 X5.3 32.09,7.18 F20.2
IN10-U
  Bottom 0.305: RN3.3 RN2.6 33.26,13.57 32.98,13.29 31.44,13.29 31.02,12.87 D7.1
  Bottom 0.813: D7.1 30.48,12.37 F20.1
IN11-D
  Bottom 0.305: RN3.5 32.45,19.19 IC1.8
IN11-R
  Bottom 0.813: JP5.4 27.66,4.35 X5.4 28.59,7.62 F21.2
IN11-U
  Bottom 0.305: RN3.4 RN2.5 32.29,13.97 29.53,13.97 28.58,13.02 D7.2
  Bottom 0.813: F21.1 D7.2
IN12-D
  Bottom 0.305: RN4.8 21.2,17.63 29.76,17.63 IC1.9
IN12-R
  Bottom 0.813: JP5.5 25.12,5.25 X5.5 25.09,7.62 F22.2
IN12-U
  Bottom 0.305: D8.1 25.08,13.02 24.13,13.97 21.05,13.97 RN1.8 RN4.1
  Bottom 0.813: F22.1 D8.1
IN13-D
  Bottom 0.305: RN4.7 20.09,18.18 20.32,18.41 29.42,18.41 IC1.10
IN13-R
  Bottom 0.813: JP5.6 22.58,4.29 X5.6 F23.2
IN13-U
  Bottom 0.305: D8.2 22.63,12.87 22.21,13.29 20.36,13.29 20.09,13.57 RN1.7 RN4.2
  Bottom 0.813: D8.2 23.18,12.37 F23.1
IN14-D
  Bottom 0.305: IC1.14 31.11,24.64 31.11,21.27 28.89,19.05 20,19.05 19.29,18.33 RN4.6
IN14-R
  Bottom 0.813: JP5.7 20.04,3.33 X5.7 F24.2
IN14-U
  Bottom 0.305: D9.1 16.74,12.87 17.16,13.29 19,13.29 19.29,13.57 RN1.6 RN4.3
  Bottom 0.813: D9.1 16.19,12.69 F24.1
IN15-D
  Bottom 0.305: IC1.15 31.45,25.94 30.56,25.05 30.56,21.98 28.26,19.68 19.68,19.68 18.48,18.48 RN4.5
IN15-R
  Bottom 0.813: JP5.8 14.72,5.28 X5.8 14.61,5.29 F25.2
IN15-U
  Bottom 0.305: D9.2 14.29,13.02 15.24,13.97 18.32,13.97 RN1.5 RN4.4
  Bottom 0.813: F25.1 14.29,11.1 D9.2
LED_BLUE  (via drill 0.35)
  Top 0.305: v39.05,26.67 40.96,26.67 45.4,22.23 R3.2
  Bottom 0.305: IC1.18 32.33,28.89 36.83,28.89 v39.05,26.67
LED_GREEN  (via drill 0.35)
  Top 0.305: v39.05,24.13 41.59,24.13 45.4,20.32 51.63,20.32 53.44,18.51 54.17,17.78 R5.2
  Bottom 0.305: IC1.16 31.04,26.67 31.83,27.45 35.73,27.45 v39.05,24.13
LED_RED  (via drill 0.35)
  Top 0.305: v39.05,25.34 39.11,25.4 41.27,25.4 45.4,21.27 53.53,21.27 R4.2
  Bottom 0.305: v39.05,25.34 36.14,28.26 31.84,28.26 IC1.17
N$11  (via drill 0.6)
  Top 0.813: v76.52,39.69 78.11,41.27 87,41.27 88.27,40.01 v90.81,40.01
  Bottom 0.813: C16.1 75.72,40.48 v76.52,39.69 | D4.3 74.81,41.92 C16.1 | IC5.10 73.38,38.66 C16.1 | v90.81,40.01 90.75,39.95 TH2.2
N$37  (via drill 0.6)
  Top 0.813: IC4.10 26.67,38.01 26.67,36.2 25.4,34.92 v7.62,34.92 5.08,34.92 3.17,33.02 3.17,26.67 v6.99,22.86
  Bottom 0.406: C14.1 3.93,34.92
  Bottom 0.61: 3.81,34.92 3.93,34.92
  Bottom 0.813: 3.93,34.92 v7.62,34.92 | 3.81,34.92 3.17,34.92 2.86,34.61 D3.3 | v6.99,22.86 TH1.2
N$46
  Bottom 0.406: R8.2 C15.1 1.91,27.62 2.22,27.94 3.81,27.94 | TH1.3 9.29,27.55 8.89,27.94 3.81,27.94 | D3.1 3.81,27.94
N$56  (via drill 0.35)
  Top 0.406: v73.03,43.81 85.72,43.81 88.44,41.1 91.61,41.1 v93.34,39.37
  Bottom 0.406: R9.2 C17.1 73.78,45.59 | D4.1 73.86,45.29 73.03,44.45 v73.03,43.81 | TH2.3 93.34,37.72 v93.34,39.37
  Bottom 0.813: 73.78,45.59 D4.1
N$57
  Bottom 0.305: R2.2 98.91,27.62
  Bottom 1.016: 98.91,27.62 D2.1 | TH3.3 99.94,31.99 98.24,30.29 C13.1 R2.2
N$60
  Top 0.305: R4.1 LED2.A
N$61
  Top 0.305: LED1.A R5.1
N$64
  Top 0.305: R3.1 LED3.A
N$70  (via drill 0.6)
  Top 0.305: v16.51,15.24 16.45,15.18
  Top 0.813: v8.89,12.06 13.34,12.06 16.45,15.18 | v16.51,15.24 v26.99,15.24 v36.51,15.24
  Bottom 0.406: C18.1 4.25,11.09 4.45,11.28
  Bottom 0.813: v36.51,15.24 38.1,15.24 D6.3 | D7.3 29.36,15.24 v26.99,15.24 24.3,15.24 D8.3 | v16.51,15.24 15.41,15.24 D9.3 | D5.3 4.45,11.28 6.64,11.28 7.43,12.06 v8.89,12.06 9.53,12.7 TH4.2
N$71  (via drill 0.35)
  Top 0.406: v3.17,16.19 8.89,16.19 v11.75,13.34
  Bottom 0.406: R6.2 2.1,13.61 | C19.2 2.1,18.41 R6.2 | R6.2 v3.17,16.19 | v11.75,13.34 11.75,15.14 TH4.3
  Bottom 0.813: 2.1,13.61 D5.1
N$80  (via drill 0.6)
  Top 0.813: v49.21,15.24 v59.05,15.24 v68.58,15.24 | v83.19,11.43 75.56,11.43 74.3,12.7 v74.37,12.7
  Bottom 0.813: D12.3 61.74,15.24 v59.05,15.24 56.69,15.24 D13.3 | v49.21,15.24 48.11,15.24 D14.3 | v68.58,15.24 68.75,15.07 D11.3 74.02,15.07 C20.1 74.37,14.49 v74.37,12.7 D10.3 | TH5.2 83.09,11.53 v83.19,11.43
N$81
  Bottom 0.305: 76.68,7.89 C21.1 | 78.38,12.34 78.42,12.38
  Bottom 0.406: R7.2 76.68,7.89 | 78.38,12.34 78.11,12.34 77.84,12.34 D10.1 | C21.1 78.42,9.72 78.42,12.38 78.42,12.92 79.33,13.82 TH5.3
N$82  (via drill 3.2 pad 5)
  other vias: 3,4
N$83  (via drill 3.2 pad 5)
  other vias: 103,4
N$84  (via drill 3.2 pad 5)
  other vias: 3,47
N$85  (via drill 3.2 pad 5)
  other vias: 103,47
OUT0-D
  Bottom 0.305: IC4.1 6.45,31.21 11.43,36.2 27.3,36.2 29.27,38.16 38.74,38.16 39.21,37.7 IC1.32
OUT0-R
  Bottom 0.813: JP3.1 12.66,49.26 X3.1 9.65,46.48 6.42,43.25 F2.2
OUT0-U
  Bottom 0.813: F2.1 6.45,38.49 IC4.18
OUT1-D
  Bottom 0.305: IC4.2 8.99,31.21 13.34,35.56 27.62,35.56 29.66,37.59 38.18,37.59 38.64,37.13 IC1.31
OUT1-R
  Bottom 0.813: JP3.2 13.45,46.48 X3.2 10.15,43.25 F3.2
OUT2-D
  Bottom 0.305: IC4.3 11.53,31.21 15.24,34.92 27.94,34.92 30.04,37.03 37.61,37.03 38.07,36.57 IC1.30
OUT2-R
  Bottom 0.813: JP3.3 16.88,47.37 X3.3 13.65,43.25 F4.2
OUT2-U
  Bottom 0.813: F4.1 11.53,40.39 IC4.16
OUT3-D
  Bottom 0.305: IC4.4 14.07,31.21 17.14,34.29 28.26,34.29 30.43,36.46 37.05,36.46 37.51,36 IC1.29
OUT3-R
  Bottom 0.813: JP3.4 21.31,47.99 20.38,47.06 X3.4 17.15,43.25 F5.2
OUT3-U
  Bottom 0.813: F5.1 14.21,38.26 IC4.15
OUT4-D
  Bottom 0.305: IC4.5 16.61,31.21 19.05,33.66 28.57,33.66 30.82,35.9 36.48,35.9 36.94,35.44 IC1.28
OUT4-R
  Bottom 0.813: JP3.5 23.88,49.23 X3.5 20.65,43.25 F6.2
OUT4-U
  Bottom 0.813: F6.1 16.61,40.1 IC4.14
OUT5-D
  Bottom 0.305: IC4.6 19.15,31.21 20.95,33.02 28.89,33.02 31.2,35.33 35.92,35.33 36.38,34.87 IC1.27
OUT5-R
  Bottom 0.813: JP3.6 26.39,47.47 X3.6 24.15,43.25 F7.2
OUT5-U
  Bottom 0.813: F7.1 19.15,39.15 IC4.13
OUT6-D
  Bottom 0.305: IC4.7 21.69,31.21 22.86,32.38 29.21,32.38 31.59,34.76 35.35,34.76 35.81,34.3 IC1.26
OUT6-R
  Bottom 0.813: JP3.7 28.93,48.42 X3.7 27.65,43.25 F8.2
OUT6-U
  Bottom 0.813: F8.1 21.69,38.2 IC4.12
OUT7-D  (via drill 0.35)
  Top 0.305: IC4.8 24.23,31.85 25.08,32.7 v36.51,32.7
  Bottom 0.305: v36.51,32.7 35.48,33.74 IC1.25
OUT7-R
  Bottom 0.813: JP3.8 31.59,49.26 X3.8 31.15,43.25 F9.2
OUT7-U
  Bottom 0.813: F9.1 27.23,41.2 24.23,38.2 IC4.11
OUT8-D
  Bottom 0.305: IC1.42 47.46,33.07 48.69,33.07 49.69,32.07 52.07,32.07 53.05,31.08 IC5.1
OUT8-R
  Bottom 0.813: JP4.1 45.04,49.26 X4.1 45.8,42.94 F10.2
OUT8-U
  Bottom 0.813: F10.1 50.8,38.42 52.75,38.42 IC5.18
OUT9-D
  Bottom 0.305: IC5.2 55.59,32.21 54.96,32.84 50.02,32.84 49.23,33.64 46.91,33.64 IC1.41
OUT9-R
  Bottom 0.813: JP4.2 48.54,49.26 X4.2 49.3,42.94 F11.2
OUT9-U  (via drill 0.6)
  Top 0.813: IC5.17 55.59,39.66 53.98,41.27 v53.66,41.27
  Bottom 0.813: F11.1 52.4,41.27 v53.66,41.27
OUT10-D
  Bottom 0.305: IC5.3 58.13,31.5 56.23,33.4 50.42,33.4 49.62,34.2 46.33,34.2 IC1.40
OUT10-R
  Bottom 0.813: JP4.3 51.15,48.37 X4.3 52.8,42.94 F12.2
OUT10-U
  Bottom 0.813: IC5.16 58.13,38.74 56.04,40.84 F12.1
OUT11-D
  Bottom 0.305: IC5.4 60.67,31.4 58.12,33.96 50.81,33.96 50,34.77 45.77,34.77 IC1.39
OUT11-R
  Bottom 0.813: JP4.4 53.69,47.41 X4.4 56.3,42.94 F13.2
OUT11-U
  Bottom 0.813: IC5.15 60.67,39.02 F13.1 | F13.1
OUT12-D
  Bottom 0.305: IC5.5 63.22,31.4 60.1,34.52 51.21,34.52 50.4,35.33 45.2,35.33 IC1.38
OUT12-R
  Bottom 0.813: JP4.5 56.23,46.51 X4.5 59.8,42.94 F14.2
OUT12-U
  Bottom 0.813: F14.1 63.22,39.97 IC5.14
OUT13-D
  Bottom 0.305: IC5.6 65.75,31.4 62.08,35.08 51.6,35.08 50.78,35.9 44.64,35.9 IC1.37
OUT13-R
  Bottom 0.813: JP4.6 58.77,47.47 X4.6 63.3,42.94 F15.2
OUT13-U
  Bottom 0.813: F15.1 65.75,40.66 IC5.13
OUT14-D
  Bottom 0.305: IC5.7 68.3,31.4 64.06,35.64 51.99,35.64 51.17,36.46 44.07,36.46 IC1.36
OUT14-R
  Bottom 0.813: JP4.7 61.31,48.42 X4.7 66.8,42.94 F16.2
OUT14-U
  Bottom 0.813: F16.1 68.3,39.71 IC5.12
OUT15-D
  Bottom 0.305: IC5.8 70.83,31.4 66.04,36.2 52.39,36.2 51.44,37.15 43.62,37.15 IC1.35
OUT15-R
  Bottom 0.813: JP4.8 63.98,49.26 X4.8 70.3,42.94 F17.2
OUT15-U
  Bottom 0.813: F17.1 72.84,40.12 IC5.11
OUT-1U
  Bottom 0.813: F3.1 8.99,39.44 IC4.17
RS-A
  Top 0.61: IC2.6 93.98,27.94 93.98,15.24 85.01,6.27 X2A.2
  Bottom 0.61: X1A.1 83.82,46.35 IC2.6
RS-B
  Top 0.61: IC2.7 92.71,26.67 92.71,15.88 81.6,4.76 X2A.1
  Bottom 0.61: X1A.2 81.28,45.8 IC2.7
RS-D  (via drill 0.35)
  Top 0.305: v36.83,18.41 27.94,18.41 24.77,21.59 24.77,24.85 JPROG.1
  Top 0.406: IC2.4 81.28,35.56 50.16,35.56 48.26,33.66 43.18,33.66 v42.55,33.02
  Bottom 0.305: IC1.3 37.34,18.41 v36.83,18.41
  Bottom 0.406: v42.55,33.02 42.55,23.62 IC1.3
RS-E  (via drill 0.35)
  Top 0.406: IC2.3 IC2.2 81.28,33.02 80.01,34.29 50.48,34.29 48.9,32.7 44.13,32.7 v41.27,29.84
  Bottom 0.406: IC1.4 41.27,23.48 v41.27,29.84 | R10.2 78.74,33.02 IC2.2
RS-R  (via drill 0.35)
  Top 0.305: JPROG.4 23.38,21.71 27.62,17.46 v36.83,17.46
  Top 0.406: IC2.1 76.2,33.02 50.8,33.02 49.53,31.75 v45.09,31.75
  Bottom 0.305: IC1.2 37.52,17.46 v36.83,17.46
  Bottom 0.406: IC1.2 45.09,25.03 v45.09,31.75
RST
  Bottom 0.305: IC1.20 32.06,31.43 30.48,31.43 27.62,28.57 22.54,28.57 20.84,26.87 JPROG.5 19.27,24.43 19.27,21.57 R1.1
SCK  (via drill 0.35)
  Top 0.305: JPROG.3 25,27.62 26.67,27.62 29.21,25.08 v34.92,25.08
  Bottom 0.305: v34.92,25.08 34.92,25.05 IC1.11
XTAL1  (via drill 0.35)
  Top 0.305: v33.97,33.97 33.97,34.49 Q1.1 38.42,38.94 v38.42,39.69
  Bottom 0.305: IC1.24 34.77,33.17 v33.97,33.97 | v38.42,39.69 36.72,39.69 C2.2
XTAL2  (via drill 0.35)
  Top 0.305: Q1.2 44.72,35.83 | 44.72,35.83 42.55,38 v42.55,39.69 | v38.73,31.75 39.37,32.38 40.64,32.38 44.08,35.83 44.72,35.83
  Bottom 0.305: v42.55,39.69 44.12,39.69 C1.1 | IC1.23 35.13,31.75 v38.73,31.75

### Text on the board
tPlace: -R | +R | 0 | 1 | 2 | 3 | 4 | 5 | 6 | 7 | ⏚ | 8 | 9 | A | B | C | D | E | F | ⏚ | GND | +12V | ↓OUTPUTS↓ | MTB-UNI v4.2 | 1 | 2 | 4 | 8 | 16 | 32 | 64 | 128 | RED | RČ&JH / 2020/21 | RST | SCK | MISO | GREEN | GND | MOSI | +5V | BLUE | KMŽ / Brno I | ↑INPUTS↑ | ↑INPUTS↑ | + 12V | LRKV / MENDELU | GND | ⏚ | F | E | D | C | B | A | 9 | 8 | ⏚ | 7 | 6 | 5 | 4 | 3 | 2 | 1 | 0 | -R | +R
tNames: ⏚ | ⏚ | ⏚ | RS485 driver must / be removed for ISP | ⏚ | ⏚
